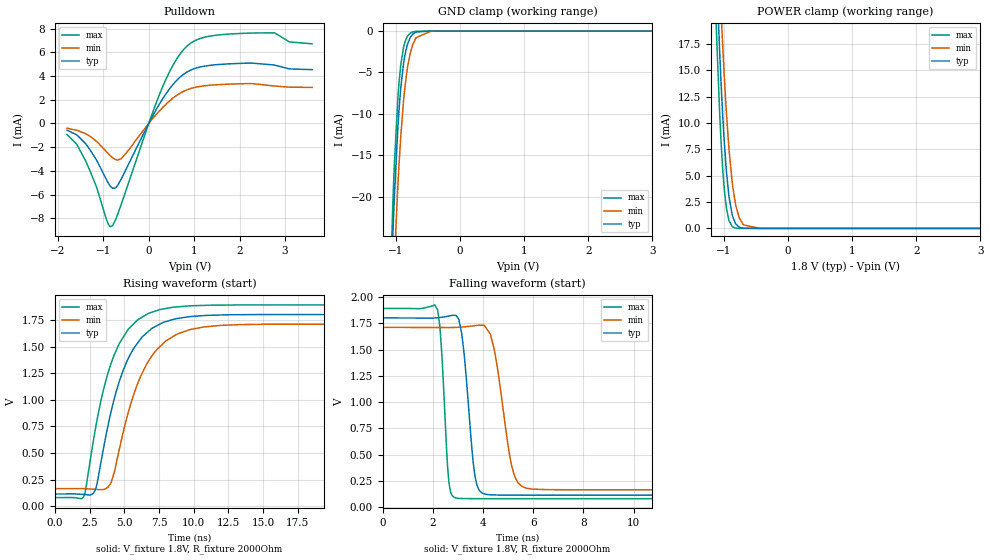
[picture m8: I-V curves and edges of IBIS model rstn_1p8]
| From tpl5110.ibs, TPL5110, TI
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|   Model
[Model]   rstn_1p8
Model_type   I/O_open_drain
Polarity   Non-Inverting
Enable   Active-Low
Vinl = 0.54
Vinh = 1.26
Vmeas = 0.9
Vref = 1.8
Cref = 1pF
Rref = 2000
|   typ   min   max
C_comp   0.474pF   0.343pF   0.582pF
[Voltage Range]   1.8   1.71   1.89
[Temperature Range]   25   105   -40
[Pullup Reference]   1.8   1.71   1.89
[Pulldown Reference]   0   0   0
[Power Clamp Reference]   1.8   1.71   1.89
[GND Clamp Reference]   0   0   0
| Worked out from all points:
|   slope of the pulldown table from 0 to 0.27 V, typ, clamps not added: 146 ohm
|   GND clamp passes 1 mA (typ) near -0.78 V on its own axis
|   POWER clamp passes 1 mA (typ) near -0.85 V on its own axis
|   falling waveform, V_fixture 1.8V, R_fixture 2000Ohm: 20-80 % time 355ps typ, 556ps min, 237ps max; typ from 1.8 V to 0.117 V
|   rising waveform, V_fixture 1.8V, R_fixture 2000Ohm: 20-80 % time 2.22ns typ, 2.39ns min, 2.08ns max; typ from 0.117 V to 1.8 V
[Pulldown]
|   Voltage   I(typ)   I(min)   I(max)
-1.8V     -571.7uA   -401.9uA   -935.3uA
-1.4V     -1.662mA   -848.3uA   -3.082mA
-844.2mV  -5.304mA   -2.734mA   -8.704mA
-736.2mV  -5.445mA   -3.037mA   -8.172mA
-606.6mV  -4.699mA   -2.977mA   -6.83mA
311.4mV   2.105mA    1.368mA    3.141mA
613.8mV   3.626mA    2.365mA    5.434mA
846mV     4.347mA    2.844mA    6.537mA
1.294V    4.876mA    3.205mA    7.332mA
2.261V    5.097mA    3.369mA    7.63mA
2.768V    4.932mA    3.159mA    7.649mA
3.6V      4.541mA    3.04mA     6.718mA
[GND Clamp]
|   Voltage   I(typ)   I(min)   I(max)
-1.8V     -271.2mA   -257.5mA   -290.2mA
-1.152V   -51.07mA   -57.26mA   -49.44mA
-1.044V   -24.77mA   -32.5mA    -20.92mA
-1.039V   -23.68mA   -31.42mA   -19.79mA
-1.017V   -19.58mA   -27.29mA   -15.63mA
-963mV    -11.35mA   -18.33mA   -7.83mA
-919.8mV  -6.849mA   -12.7mA    -4.083mA
-849.6mV  -2.692mA   -6.394mA   -1.191mA
-768.6mV  -733.1uA   -2.559mA   -229.2uA
-682.2mV  -124.3uA   -797.2uA   -33.36uA
-444.6mV  -228.5nA   -4.654uA   -7.004nA
3.6V      0A         0A         0A
[POWER Clamp]
|   Voltage   I(typ)   I(min)   I(max)
-1.8V     177.4mA    171.8mA    183.6mA
-1.114V   24.86mA    31.59mA    18.98mA
-1.066V   17.28mA    24.18mA    11.44mA
-1.033V   12.93mA    19.7mA     7.474mA
-1.022V   11.62mA    18.31mA    6.367mA
-990mV    8.172mA    14.42mA    3.705mA
-919.8mV  3.167mA    7.757mA    813.9uA
-860.4mV  1.145mA    4.066mA    142.7uA
-811.8mV  419.7uA    2.196mA    23.16uA
-693mV    15.38uA    335.2uA    102.7nA
-444.6mV  0A         725.9nA    0A
3.6V      0A         0A         0A
[Ramp]
R_load = 2000
|   typ   min   max
dV/dt_r   1.01005/2.21985e-09   0.925593/2.39098e-09   1.08406/2.08345e-09
dV/dt_f   1.01005/3.54855e-10   0.925589/5.56051e-10   1.08406/2.36987e-10
[Falling Waveform]
V_fixture = 1.8V
V_fixture_min = 1.71V
V_fixture_max = 1.89V
R_fixture = 2000Ohm
C_fixture = 0F
|   Time   V(typ)   V(min)   V(max)
0s        1.8V       1.71V      1.89V
2.189ns   1.802V     1.709V     1.876V
2.623ns   1.817V     1.709V     275.7mV
2.945ns   1.818V     1.71V      88.96mV
3.247ns   1.452V     1.715V     84.25mV
3.702ns   266.8mV    1.727V     83.64mV
4.181ns   122.6mV    1.684V     83.29mV
5.236ns   117.1mV    312.7mV    83.29mV
5.927ns   116.7mV    175.4mV    83.28mV
50ns      116.6mV    167.4mV    83.24mV
[Rising Waveform]
V_fixture = 1.8V
V_fixture_min = 1.71V
V_fixture_max = 1.89V
R_fixture = 2000Ohm
C_fixture = 0F
|   Time   V(typ)   V(min)   V(max)
0s        116.6mV    167.3mV    83.24mV
2.068ns   113.1mV    167.8mV    87.86mV
2.927ns   156.1mV    160.4mV    728.4mV
3.837ns   761.1mV    181mV      1.253V
5.359ns   1.407V     912.4mV    1.671V
6.486ns   1.613V     1.303V     1.791V
7.564ns   1.709V     1.498V     1.847V
9.726ns   1.781V     1.659V     1.881V
13.36ns   1.798V     1.705V     1.889V
50ns      1.8V       1.71V      1.89V
